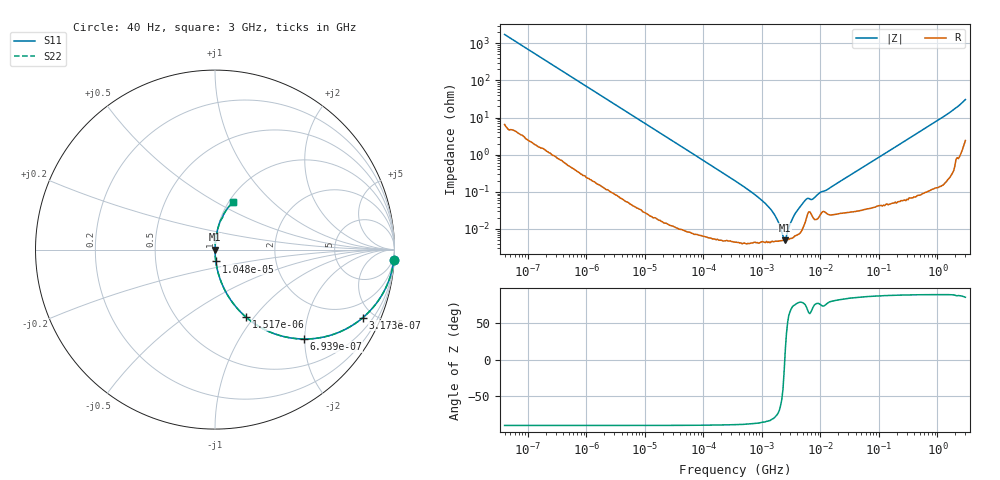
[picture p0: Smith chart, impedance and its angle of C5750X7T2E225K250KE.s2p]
! S-parameter Generated by TDK Corporation
! Copyright(C) 2015 TDK Corporation.
! All Rights Reserved.
! TDK P/N: C5750X7T2E225K250KE (Multilayer Ceramic Chip Capacitors)
! Property: C=2.2uF
! Size(LxWxT): 5.7x5x2.5mm, 0.224x0.197x0.098inches
! Model Type: s2p (Touchstone File Format Version 1.0)
! Frequency: DC=Yes Start=0.00004MHz Stop=3000MHz 396points Log-sweep
! Note: This model was converted from impedance.
! Model Generated on Jun. 23, 2015
! Hash(MD5):
! Port Assignments:
!  1 ---| |--- 2
! Applicable Conditions:
!  Temperature = 25 degC
!  DC Bias Voltage = 0 V
!  Small Signal Operation
! Terms and conditions regarding TDK Simulation Models
! (1)This simulation model is being provided solely for informational purposes. Please refer to the specifications of the products in terms of detailed characteristics of such products.
! (2)In no event shall TDK Corporation of any of its subsidiaries be liable for any loss or damage arising, directly or indirectly,
!  From any information contained in this simulation model, including, but not limited to loss or damages arising from any inaccuracies, omissions or errors in connection with such information.
! (3)Any and all copyrights on this simulation model are owned by TDK Corporation.
!  Duplication or redistribution of this simulation model without prior written permission from TDK Corporation is prohibited.
! (4)This simulation model is subject to any modification or change without any prior notice.
! (5)Neither TDK Corporation nor any of its subsidiaries shall make any warranty, express or implied,
!  Including but not limited to the correctness, implied warranties of merchantability and fitness for a particular purpose with respect to this simulation models.
! (6)The use of this simulation model shall be deemed to have consented to the terms and conditions hereof.
# MHz S MA R 50
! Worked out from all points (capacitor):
!   395 points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, 40 Hz to 3 GHz, reference 50 ohm
!   read as one part in series: C = 2.31 uF near 41.88 Hz
!   lowest |Z| = 5.01 mohm at 2.506 MHz (marker M1)
!   series resonance near 2.457 MHz, so ESL is about 1.8 nH
!   S11 on the Smith chart (normalised r, x): 40 Hz: 1, -34; 317.3 Hz: 1.02, -4.34; 693.9 Hz: 1.01, -1.99; 1.517 kHz: 1.00, -0.91; 10.48 kHz: 1.00, -0.13; 3 GHz: 1.05, +0.61
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4e-05  0.9981 -3.3  0.0579 86.5  0.0579 86.5  0.9981 -3.3
0.0001451139  0.9778 -11.9  0.2062 77.9  0.2062 77.9  0.9778 -11.9
0.0003173189  0.9071 -24.7  0.4176 65.1  0.4176 65.1  0.9071 -24.7
0.0006938775  0.7041 -45.0  0.7076 44.8  0.7076 44.8  0.7041 -45.0
0.000834128  0.6367 -50.3  0.7689 39.5  0.7689 39.5  0.6367 -50.3
0.001517294  0.4142 -65.3  0.9087 24.5  0.9087 24.5  0.4142 -65.3
0.003168613  0.2135 -77.5  0.9761 12.3  0.9761 12.3  0.2135 -77.5
0.01048439  0.06617 -86.0  0.9975 3.8  0.9975 3.8  0.06617 -86.0
0.01739424  0.03998 -87.5  0.999 2.3  0.999 2.3  0.03998 -87.5
0.3464102  0.001984 -88.6  1 0.1  1 0.1  0.001984 -88.6
1.146211  0.0004841 -84.9  1 0.0  1 0.0  0.0004841 -84.9
1.656397  0.0002365 -78.7  1 0.0  1 0.0  0.0002365 -78.7
2.084979  0.0001042 -62.4  1 0.0  1 0.0  0.0001042 -62.4
2.506407  5.006e-05 12.9  1 -0.0  1 -0.0  5.006e-05 12.9
2.877491  0.0001062 60.7  0.9999 -0.0  0.9999 -0.0  0.0001062 60.7
3.622024  0.0002459 74.9  0.9999 -0.0  0.9999 -0.0  0.0002459 74.9
5.480732  0.0005924 75.3  0.9998 -0.0  0.9998 -0.0  0.0005924 75.3
7.22376  0.0006255 69.2  0.9998 -0.0  0.9998 -0.0  0.0006255 69.2
9.969551  0.0009681 75.5  0.9998 -0.1  0.9998 -0.1  0.0009681 75.5
150.6385  0.01278 87.2  0.9995 -0.7  0.9995 -0.7  0.01278 87.2
1040.901  0.08577 84.2  0.995 -4.9  0.995 -4.9  0.08577 84.2
3000  0.2857 68.9  0.9361 -16.5  0.9361 -16.5  0.2857 68.9
